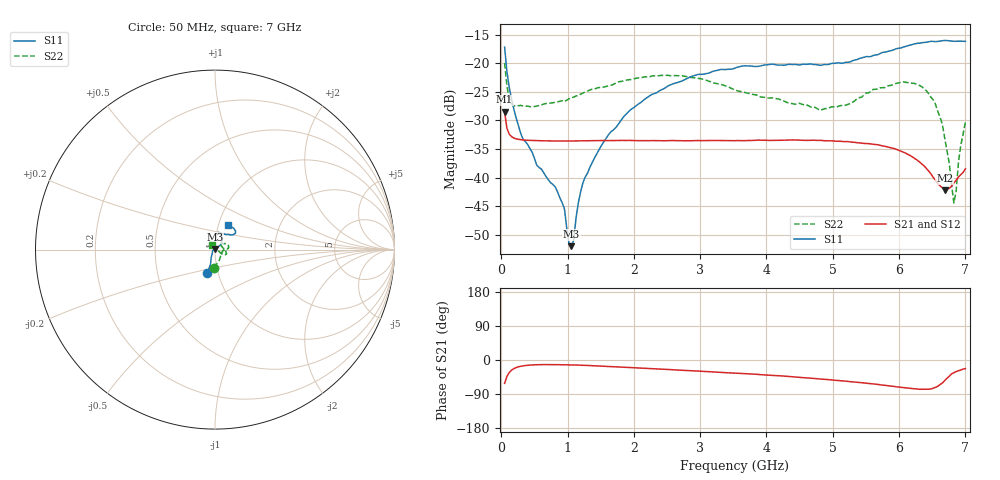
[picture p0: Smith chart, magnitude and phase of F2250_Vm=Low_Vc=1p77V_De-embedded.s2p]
! Integrated Device Technology
! Corporate Headquarters
! 6024 Silver Creek Valley Road
! San Jose, CA 95138  USA
! Phone:  1-408-284-8200
! Toll Free:  1-800-223-1366
! Webpage:  http://www.idt.com/
! Timing and RF Division
! 515 Groton Road, Suite 102
! Westford, MA 01886-6024
! Device:  F2250
! Description: Voltage Variable RF Attenuator
! Frequency:  50.0 -  6000.00 MHz
! Package:  3x3 mm Thin QFN Plastic Package: 16 pin
! Ports:  2 RF, 3 DC
!  Pin  1  = GND
!  Pin  2  = NC
!  Pin  3  = RF1  = Port 1
!  Pin  4  = NC
!  Pin  5  = GND
!  Pin  6  = GND
!  Pin  7  = GND
!  Pin  8  = GND
!  Pin  9  = NC
!  Pin 10  = RF2  = Port 2
!  Pin 11  = NC
!  Pin 12  = GND
!  Pin 13  = GND
!  Pin 14  = VCNTRL
!  Pin 15  = VDD
!  Pin 16  = VMODE
! Vcntrl:  1.770 Volts
! Vmode:  +0.000 Volts
! Vdd:  +3.30  Volts
! Current:  1.184 mA
! Data:  The device was measured on a the F2250 evaluation board which has
!  individual transmission lines to the RF pins.  Data was collected
!  using a calibrated network analyzer.  The evaluation board was
!  de-embedded using a TRL calibration technique.
!  The reference plane is the edge of the package pin.
! Misc:  SN 10
!  Action Tracker AT0258
! Date Measured:  2014-11-26
! Date:  2015-10-15  MJV
! Note:
!  Integrated Device Technology supplies this data as a sample of measured
!  data at the package pin for this product.  Your particular data for this
!  product may vary.
!  Data was taken at 25 degrees C.
!  Integrated Device Technology reserves the right to change this data at anytime.
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# GHz S dB R 50
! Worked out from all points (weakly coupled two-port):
!   201 points, 50 MHz to 7 GHz, reference 50 ohm
!   highest |S21| = -28.47 dB at 50 MHz (marker M1); lowest = -42.2 dB at 6.687 GHz (marker M2)
!   lowest |S11| = -52.0 dB at 1.058 GHz (marker M3), VSWR 1.01, Z = 49.9 + j0.228 ohm
!   |S11| at or under -10 dB: start of sweep to end of sweep
!   |S22| runs from -44.4 to -20.0 dB; largest |S21 - S12| = 7.9e-05
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0.05  -17.17 -108.3  -28.47 -61.6  -28.47 -61.6  -19.95 -92.9
0.1195  -24.20 -111.2  -32.39 -33.2  -32.38 -33.2  -26.08 -52.4
0.29325  -32.27 -126.5  -33.37 -16.5  -33.38 -16.5  -27.37 -22.1
0.84925  -42.53 170.7  -33.60 -12.3  -33.61 -12.3  -26.75 -5.9
0.9535  -45.51 170.3  -33.59 -12.6  -33.59 -12.6  -26.70 -5.2
1.023  -51.68 141.2  -33.60 -12.8  -33.60 -12.8  -26.22 -3.7
1.05775  -52.00 114.5  -33.59 -13.0  -33.59 -13.0  -26.07 -3.2
1.2315  -40.92 41.0  -33.57 -13.9  -33.56 -13.9  -25.19 -4.2
1.6485  -32.04 40.6  -33.53 -17.2  -33.52 -17.2  -23.87 1.6
2.37825  -24.87 46.8  -33.54 -23.8  -33.54 -23.8  -22.16 11.0
3.525  -20.84 72.2  -33.54 -34.6  -33.54 -34.6  -24.68 35.0
4.7065  -20.21 72.2  -33.46 -48.5  -33.47 -48.5  -27.67 43.0
5.193  -19.82 56.9  -33.70 -55.8  -33.69 -55.8  -27.34 17.6
5.85325  -17.84 40.3  -34.72 -68.3  -34.71 -68.3  -23.89 -13.6
6.3745  -16.35 41.2  -37.91 -77.3  -37.94 -77.4  -24.38 -27.4
6.54825  -16.21 45.0  -40.45 -72.1  -40.47 -72.1  -27.16 -31.7
6.68725  -16.01 48.7  -42.24 -54.4  -42.23 -54.2  -33.03 -23.3
6.75675  -16.07 51.0  -41.87 -42.9  -41.87 -42.7  -37.50 -13.7
6.82625  -16.15 53.5  -40.94 -33.4  -40.94 -33.2  -44.45 51.0
6.861  -16.14 55.0  -40.47 -30.5  -40.44 -30.4  -42.30 84.3
6.9305  -16.13 59.1  -39.50 -26.6  -39.49 -26.5  -34.37 118.2
7  -16.15 63.1  -38.47 -22.8  -38.44 -22.7  -30.26 123.0
